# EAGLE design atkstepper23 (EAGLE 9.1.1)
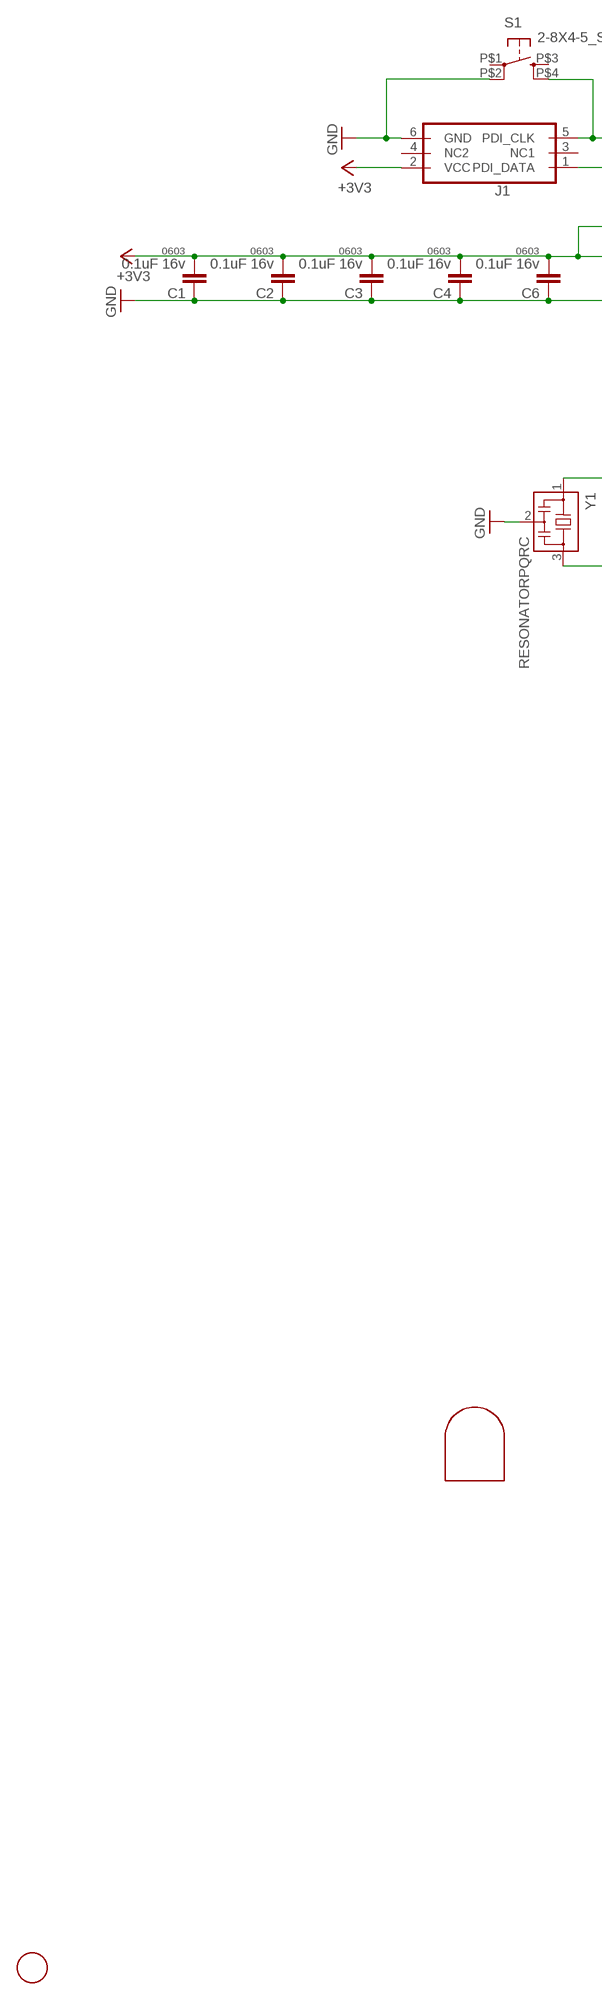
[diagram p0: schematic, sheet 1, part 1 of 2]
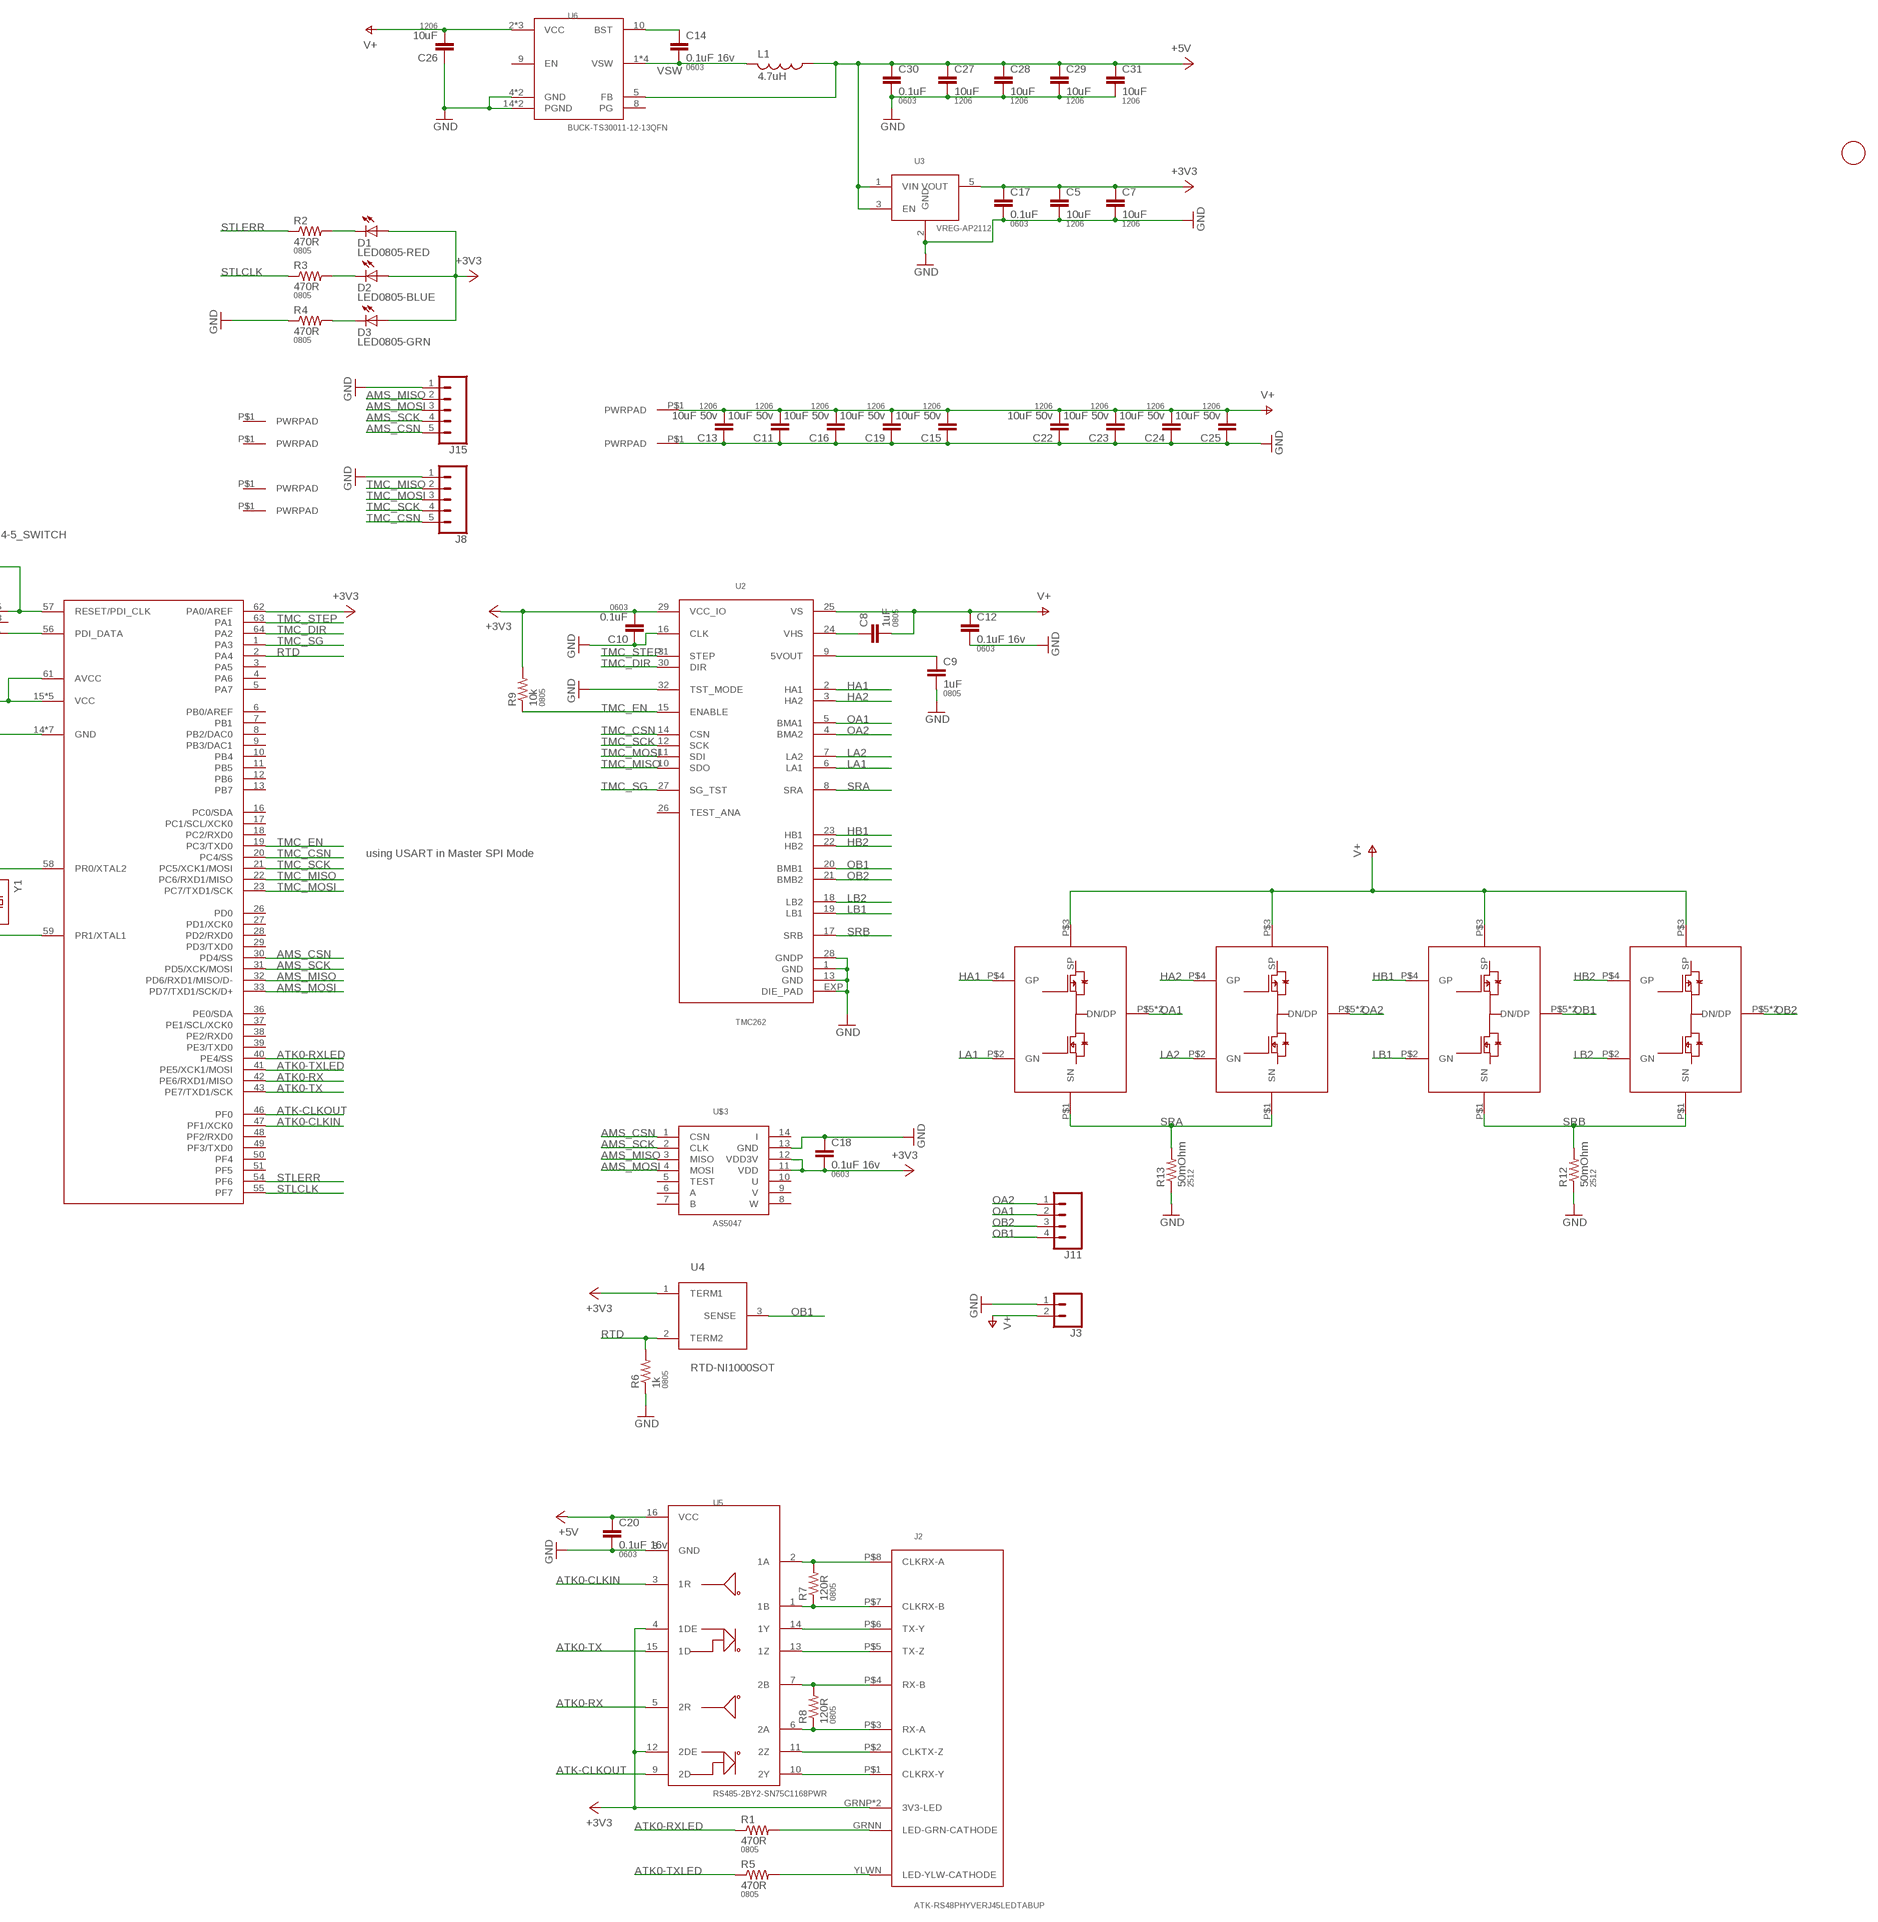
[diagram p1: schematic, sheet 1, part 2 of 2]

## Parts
C1  0.1uF 16v  CAP0603-CAP  [0603-CAP]
C2  0.1uF 16v  CAP0603-CAP  [0603-CAP]
C3  0.1uF 16v  CAP0603-CAP  [0603-CAP]
C4  0.1uF 16v  CAP0603-CAP  [0603-CAP]
C5  10uF  CAP1206  [1206]
C6  0.1uF 16v  CAP0603-CAP  [0603-CAP]
C7  10uF  CAP1206  [1206]
C8  1uF  CAP0805  [0805]
C9  1uF  CAP0805  [0805]
C10  0.1uF  CAP0603-CAP  [0603-CAP]
C11  10uF 50v  CAP1206  [1206]
C12  0.1uF 16v  CAP0603-CAP  [0603-CAP]
C13  10uF 50v  CAP1206  [1206]
C14  0.1uF 16v  CAP0603-CAP  [0603-CAP]
C15  10uF 50v  CAP1206  [1206]
C16  10uF 50v  CAP1206  [1206]
C17  0.1uF  CAP0603-CAP  [0603-CAP]
C18  0.1uF 16v  CAP0603-CAP  [0603-CAP]
C19  10uF 50v  CAP1206  [1206]
C20  0.1uF 16v  CAP0603-CAP  [0603-CAP]
C22  10uF 50v  CAP1206  [1206]
C23  10uF 50v  CAP1206  [1206]
C24  10uF 50v  CAP1206  [1206]
C25  10uF 50v  CAP1206  [1206]
C26  10uF  CAP1206  [1206]
C27  10uF  CAP1206  [1206]
C28  10uF  CAP1206  [1206]
C29  10uF  CAP1206  [1206]
C30  0.1uF  CAP0603-CAP  [0603-CAP]
C31  10uF  CAP1206  [1206]
D1  LED0805-RED  LED0805  [LED0805]
D2  LED0805-BLUE  LED0805  [LED0805]
D3  LED0805-GRN  LED0805  [LED0805]
J1  PDITHRU  [PDI_2X3_THRU]
J2  ATK-RS48PHYVERJ45LEDTABUP  [RJ45-LED-RJHSE-5381-UPTAB]
J3  CONN_02PTH3  [1X02_LONGPADS]
J4  PWRPADM3-SKINNY  [PWRPAD_3-25MM-SKINNY]
J6  PWRPADM3-SKINNY  [PWRPAD_3-25MM-SKINNY]
J8  CONN_05NO_SILK  [1X05_NO_SILK]
J9  PWRPADM3-STANDOFF  [PWRPAD_M3_STANDOFF]
J10  PWRPADM3-STANDOFF  [PWRPAD_M3_STANDOFF]
J11  CONN_04LONGPADS  [1X04_LONGPADS]
J12  PWRPADM3-SKINNY  [PWRPAD_3-25MM-SKINNY]
J13  PWRPADM3-SKINNY  [PWRPAD_3-25MM-SKINNY]
J15  CONN_05NO_SILK  [1X05_NO_SILK]
L1  4.7uH  INDUCTOR  [NRS5020T4R7MMGJ]
MP1  JRTOMBSTONE  [JRTOMBSTONE]
Q1  PNPAIR-STL40C30H3LL-FDD8424HSTM  [POWERFLAT-5X6]
Q2  PNPAIR-STL40C30H3LL-FDD8424HSTM  [POWERFLAT-5X6]
Q3  PNPAIR-STL40C30H3LL-FDD8424HSTM  [POWERFLAT-5X6]
Q4  PNPAIR-STL40C30H3LL-FDD8424HSTM  [POWERFLAT-5X6]
R1  470R  RESISTOR0805-RES  [0805]
R2  470R  RESISTOR0805-RES  [0805]
R3  470R  RESISTOR0805-RES  [0805]
R4  470R  RESISTOR0805-RES  [0805]
R5  470R  RESISTOR0805-RES  [0805]
R6  1k  RESISTOR0805-RES  [0805]
R7  120R  RESISTOR0805-RES  [0805]
R8  120R  RESISTOR0805-RES  [0805]
R9  10k  RESISTOR0805-RES  [0805]
R12  50mOhm  RESISTOR2512  [R2512]
R13  50mOhm  RESISTOR2512  [R2512]
S1  2-8X4-5_SWITCH  [TACT-SWITCH-KMR6]
U1  ATXMEGA_A3UQFN  [QFN-64-9X9MM]
U2  TMC262  [QFN32]
U3  VREG-AP2112  [SOT23-5]
U4  RTD-NI1000SOT  [SOT23]
U5  RS485-2BY2-SN75C1168PWR  [TSSOP16]
U6  BUCK-TS30011-12-13QFN  [QFN16-3X3-TI-RTE]
U$1  FIDUCIAL  [FIDUCIAL_1MM]
U$2  FIDUCIAL  [FIDUCIAL_1MM]
U$3  AS5047  [TSSOP14]
Y1  RESONATORPQRC  [RES_PRQC]

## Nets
+3V3: C1.2 C2.2 C3.2 C4.2 C5.1 C6.2 C7.1 C10.2 C17.1 C18.2 D1.1(A) D2.1(A) D3.1(A) J1.2(VCC) J2.GRNP(3V3-LED) J2.YLWP(3V3-LED) R9.2 U1.15(VCC) U1.25(VCC) U1.35(VCC) U1.45(VCC) U1.53(VCC) U1.61(AVCC) U1.62(PA0/AREF) U2.29(VCC_IO) U3.5(VOUT) U4.1(TERM1) U5.4(1DE) U5.12(2DE) U$3.11(VDD) U$3.12(VDD3V)
+5V: C20.1 C27.1 C28.1 C29.1 C30.1 C31.1 L1.1 U3.1(VIN) U3.3(EN) U5.16(VCC) U6.5(FB)
AMS_CSN: J15.5 U1.30(PD4/SS) U$3.1(CSN)
AMS_MISO: J15.2 U1.32(PD6/RXD1/MISO/D-) U$3.3(MISO)
AMS_MOSI: J15.3 U1.33(PD7/TXD1/SCK/D+) U$3.4(MOSI)
AMS_SCK: J15.4 U1.31(PD5/XCK/MOSI) U$3.2(CLK)
ATK0-CLKIN: U1.47(PF1/XCK0) U5.3(1R)
ATK0-RX: U1.42(PE6/RXD1/MISO) U5.5(2R)
ATK0-RXLED: R1.1 U1.40(PE4/SS)
ATK0-TX: U1.43(PE7/TXD1/SCK) U5.15(1D)
ATK0-TXLED: R5.1 U1.41(PE5/XCK1/MOSI)
ATK-CLKOUT: U1.46(PF0) U5.9(2D)
GND: C1.1 C2.1 C3.1 C4.1 C5.2 C6.1 C7.2 C9.2 C10.1 C11.1 C12.2 C13.1 C15.1 C16.1 C17.2 C18.1 C19.1 C20.2 C22.1 C23.1 C24.1 C25.1 C26.1 C27.2 C28.2 C29.2 C30.2 C31.2 J1.6(GND) J3.1 J8.1 J10.P$1(PWRPAD) J15.1 R4.1 R6.1 R12.1 R13.1 S1.P$2(P1) U1.14(GND) U1.24(GND) U1.34(GND) U1.44(GND) U1.52(GND) U1.60(GND) U1.P$1(GND) U2.1(GND) U2.13(GND) U2.16(CLK) U2.28(GNDP) U2.32(TST_MODE) U2.EXP(DIE_PAD) U3.2(GND) U5.8(GND) U6.4(GND) U6.14(PGND) U6.15(PGND) U6.TH(GND) U$3.13(GND) Y1.2
HA1: Q1.P$4(GP) U2.2(HA1)
HA2: Q2.P$4(GP) U2.3(HA2)
HB1: Q3.P$4(GP) U2.23(HB1)
HB2: Q4.P$4(GP) U2.22(HB2)
LA1: Q1.P$2(GN) U2.6(LA1)
LA2: Q2.P$2(GN) U2.7(LA2)
LB1: Q3.P$2(GN) U2.19(LB1)
LB2: Q4.P$2(GN) U2.18(LB2)
N$1: D3.2(C) R4.2
N$2: C8.1 U2.24(VHS)
N$3: J2.P$8(CLKRX-A) R7.2 U5.2(1A)
N$4: J1.5(PDI_CLK) S1.P$4(S1) U1.57(RESET/PDI_CLK)
N$5: D2.2(C) R3.2
N$6: D1.2(C) R2.2
N$7: U1.58(PR0/XTAL2) Y1.1
N$8: U1.59(PR1/XTAL1) Y1.3
N$10: J1.1(PDI_DATA) U1.56(PDI_DATA)
N$11: J2.P$7(CLKRX-B) R7.1 U5.1(1B)
N$12: J2.P$6(TX-Y) U5.14(1Y)
N$13: J2.P$5(TX-Z) U5.13(1Z)
N$14: J2.P$4(RX-B) R8.2 U5.7(2B)
N$15: J2.P$3(RX-A) R8.1 U5.6(2A)
N$16: J2.P$2(CLKTX-Z) U5.11(2Z)
N$17: J2.P$1(CLKRX-Y) U5.10(2Y)
N$18: C9.1 U2.9(5VOUT)
N$19: J2.GRNN(LED-GRN-CATHODE) R1.2
N$20: J2.YLWN(LED-YLW-CATHODE) R5.2
N$23: C14.1 U6.10(BST)
OA1: J11.2 Q1.P$5(DN/DP) Q1.P$8(DN/DP) U2.5(BMA1)
OA2: J11.1 Q2.P$5(DN/DP) Q2.P$8(DN/DP) U2.4(BMA2)
OB1: J11.4 Q3.P$5(DN/DP) Q3.P$8(DN/DP) U2.20(BMB1) U4.3(SENSE)
OB2: J11.3 Q4.P$5(DN/DP) Q4.P$8(DN/DP) U2.21(BMB2)
RTD: R6.2 U1.2(PA4) U4.2(TERM2)
SRA: Q1.P$1(SN) Q2.P$1(SN) R13.2 U2.8(SRA)
SRB: Q3.P$1(SN) Q4.P$1(SN) R12.2 U2.17(SRB)
STLCLK: R3.1 U1.55(PF7)
STLERR: R2.1 U1.54(PF6)
TMC_CSN: J8.5 U1.20(PC4/SS) U2.14(CSN)
TMC_DIR: U1.64(PA2) U2.30(DIR)
TMC_EN: R9.1 U1.19(PC3/TXD0) U2.15(ENABLE)
TMC_MISO: J8.2 U1.22(PC6/RXD1/MISO) U2.10(SDO)
TMC_MOSI: J8.3 U1.23(PC7/TXD1/SCK) U2.11(SDI)
TMC_SCK: J8.4 U1.21(PC5/XCK1/MOSI) U2.12(SCK)
TMC_SG: U1.1(PA3) U2.27(SG_TST)
TMC_STEP: U1.63(PA1) U2.31(STEP)
V+: C8.2 C11.2 C12.1 C13.2 C15.2 C16.2 C19.2 C22.2 C23.2 C24.2 C25.2 C26.2 J3.2 J9.P$1(PWRPAD) Q1.P$3(SP) Q2.P$3(SP) Q3.P$3(SP) Q4.P$3(SP) U2.25(VS) U6.2(VCC) U6.3(VCC) U6.11(VCC)
VSW: C14.2 L1.2 U6.1(VSW) U6.12(VSW) U6.13(VSW) U6.16(VSW)
Unconnected: J1.3(NC1) J1.4(NC2) J4.P$1(PWRPAD) J6.P$1(PWRPAD) J12.P$1(PWRPAD) J13.P$1(PWRPAD) S1.P$1(P) S1.P$3(S) U1.3(PA5) U1.4(PA6) U1.5(PA7) U1.6(PB0/AREF) U1.7(PB1) U1.8(PB2/DAC0) U1.9(PB3/DAC1) U1.10(PB4) U1.11(PB5) U1.12(PB6) U1.13(PB7) U1.16(PC0/SDA) U1.17(PC1/SCL/XCK0) U1.18(PC2/RXD0) U1.26(PD0) U1.27(PD1/XCK0) U1.28(PD2/RXD0) U1.29(PD3/TXD0) U1.36(PE0/SDA) U1.37(PE1/SCL/XCK0) U1.38(PE2/RXD0) U1.39(PE3/TXD0) U1.48(PF2/RXD0) U1.49(PF3/TXD0) U1.50(PF4) U1.51(PF5) U2.26(TEST_ANA) U6.8(PG) U6.9(EN) U$3.5(TEST) U$3.6(A) U$3.7(B) U$3.8(W) U$3.9(V) U$3.10(U) U$3.14(I)

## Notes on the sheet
- using USART in Master SPI Mode

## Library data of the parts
C1-C4 C6 C10 C12 C14 C17 C18 C20 C30 = borkedlabs-passives:CAP: Capacitor; PACKAGE: 0603
C5 C7 C11 C13 C15 C16 C19 C22-C29 C31 = borkedlabs-passives:CAP: Capacitor; PACKAGE: 1206
C8 C9 = borkedlabs-passives:CAP: Capacitor; PACKAGE: 0805
D1-D3 = lights:LED: LED
J1 = microcontrollers:PDI: Multi connection point. Often used as Generic Header-pin footprint for 0.1 inch spaced/style header connections You can populate with any combo of single row headers, but if you'd like an exact match, check these: Header - 2x3 (Male, 0.1") (PRT-12807) Header - 2x3 (Female, 0.1") (PRT-13010) 2x3 Pin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
J2 = connector:ATK-RS48PHYVE
J3 = SparkFun-Connectors:CONN_02: Multi connection point. Often used as Generic Header-pin footprint for 0.1 inch spaced/style header connections
J4 J6 J9 J10 J12 J13 = power:PWRPAD
J8 J15 = SparkFun-Connectors:CONN_05: Multi connection point. Often used as Generic Header-pin footprint for 0.1 inch spaced/style header connections On any of the 0.1 inch spaced packages, you can populate with these: Break Away Headers - Straight (PRT-00116) Break Away Male Headers - Right Angle (PRT-00553) Female Headers (PRT-00115)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
J11 = SparkFun-Connectors:CONN_04: Multi connection point. Often used as Generic Header-pin footprint for 0.1 inch spaced/style header connections On any of the 0.1 inch spaced packages, you can populate with these: Break Away Headers - Straight (PRT-00116) Break Away Male Headers - Right Angle (PRT-00553) Female Headers (PRT-00115)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; PROD_ID: CONN-09696
L1 = power:INDUCTOR
MP1 = connector:JRTOMBSTONE
Q1-Q4 = power:PNPAIR-STL40C30H3LL-FDD8424H
R1-R9 = borkedlabs-passives:RESISTOR: Resistor; PACKAGE: 0805
R12 R13 = borkedlabs-passives:RESISTOR: Resistor; PACKAGE: 2512
S1 = fab:2-8X4-5_SWITCH
U1 = microcontrollers:ATXMEGA_A3U
U2 = power:TMC262
U3 = power:VREG-AP2112
U4 = sensor:RTD-NI1000SOT
U5 = comm:RS485-2BY2-SN75C1168PWR
U6 = power:BUCK-TS30011-12-13
U$1 U$2 = connector:FIDUCIAL: For use by pick and place machines to calibrate the vision/machine, 1mm
U$3 = sensor:AS5047
Y1 = passives:RESONATOR

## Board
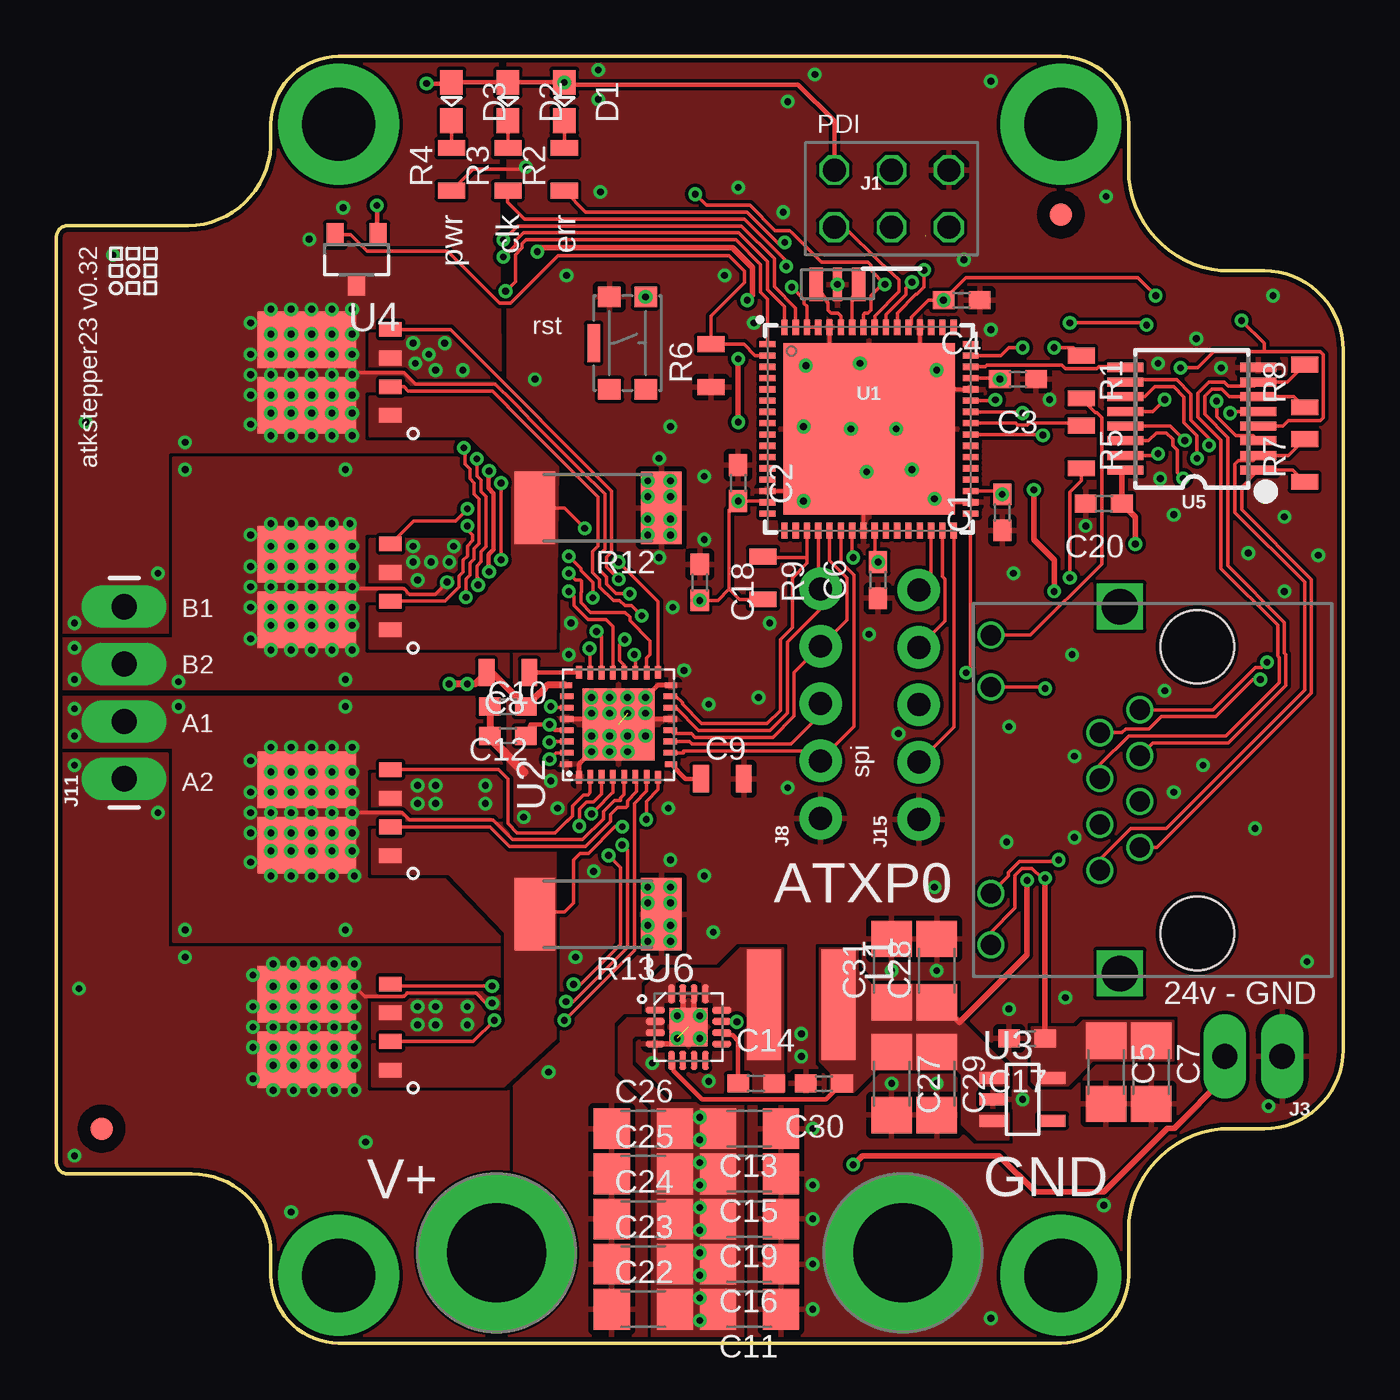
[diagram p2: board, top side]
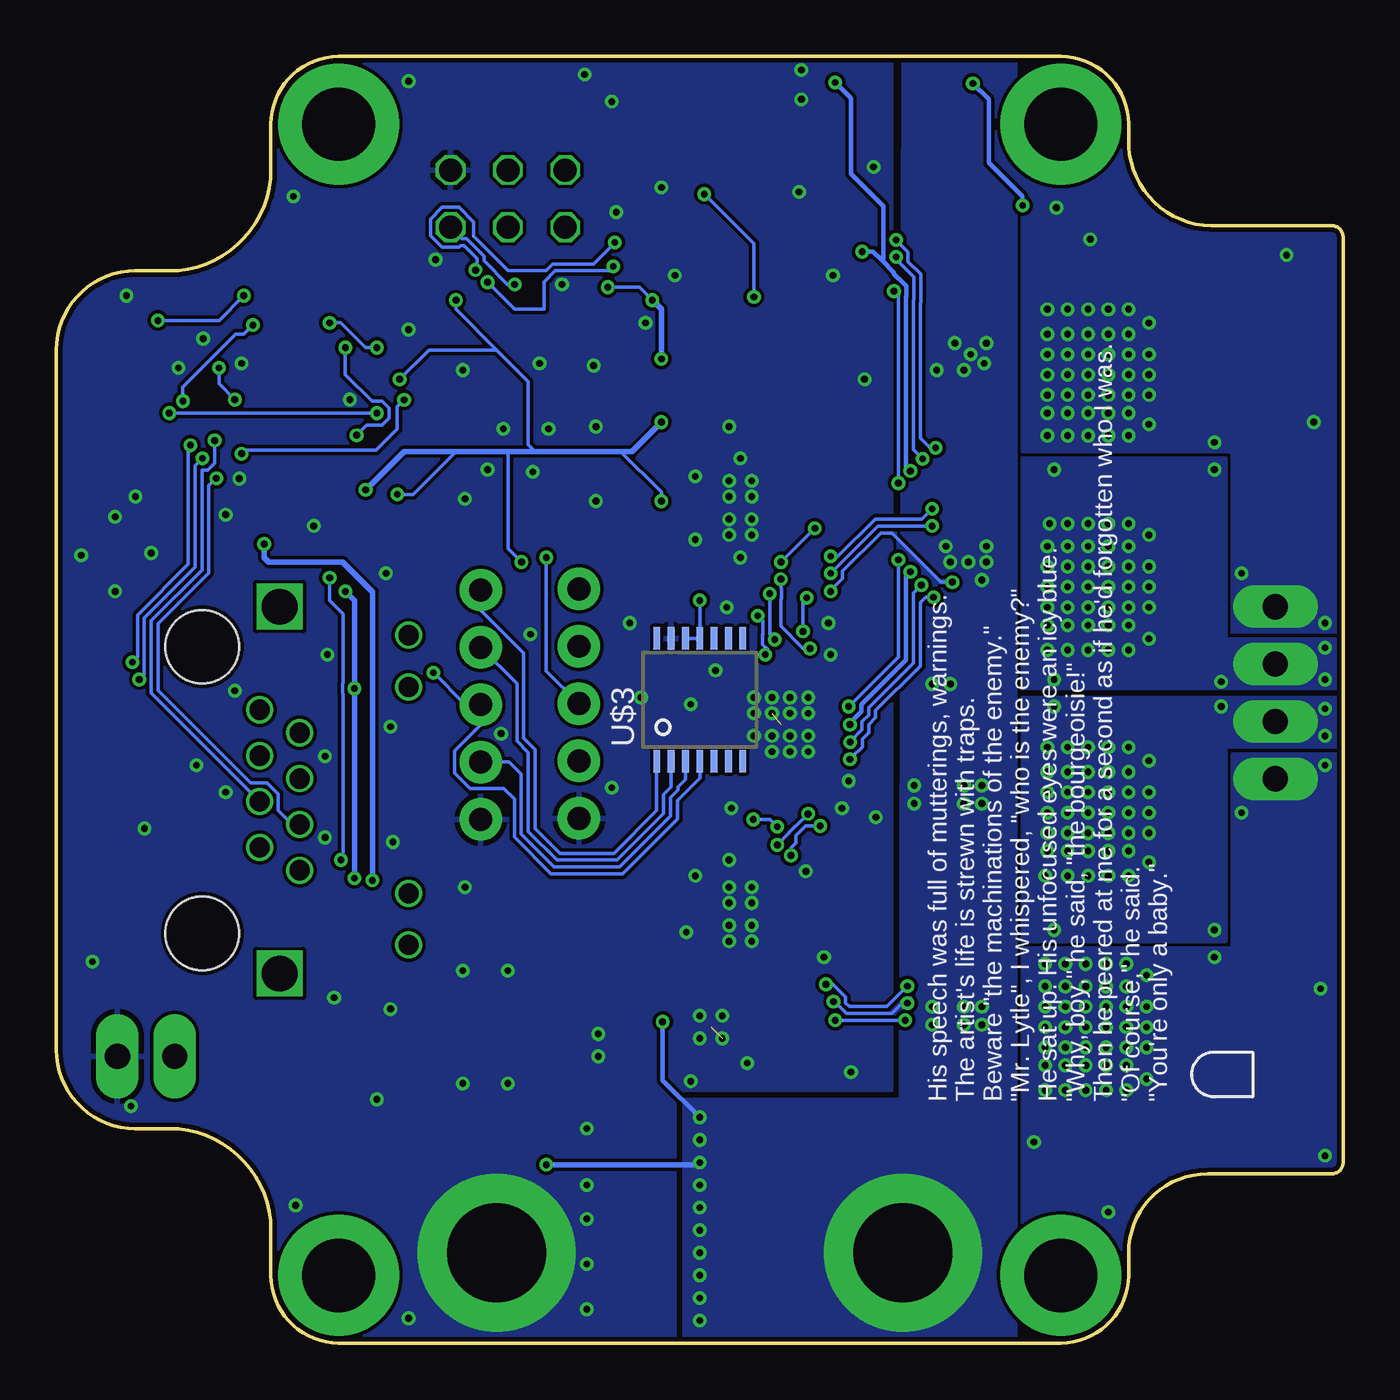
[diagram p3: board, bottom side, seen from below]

Size 57 x 57 mm. Coordinates in mm from the lower left corner, seen from the top.
Outline: 44.5,0 12.5,0 arc-90 9.5,3 9.5,4 arc90 6,7.5 0.5,7.5 arc-90 0,8 0,49 arc-90 0.5,49.5 5.5,49.5 arc90 9.5,53 9.5,54 arc-90 12.5,57 44.5,57 arc-90 47.5,54 47.5,52 arc90 52,47.5 53.5,47.5 arc-90 57,44 57,13 arc-90 53.5,9.5 52,9.5 arc90 47.5,5 47.5,3 arc-90 44.5,0
Copper layers (1*16): Top 0.035mm / dielectric 1.5mm / Bottom 0.035mm
Design rules "default *": minimum track width 6mil, minimum drill 0.3mm, track to track 6mil, track to pad 6mil, pad to pad 6mil, via to via 6mil, smd to smd 6mil, copper to edge 8mil, drill to drill 8mil, minimum pad ring 6mil, minimum via ring 6mil, stop-mask expansion 4mil, vias tented up to drill 27mil, thermal gap 9mil

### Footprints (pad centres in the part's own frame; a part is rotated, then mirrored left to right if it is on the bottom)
0603-CAP = smd 0.96 x 0.8: 1 -0.8,0; 2 0.8,0
1206 = smd 1.6 x 1.8: 1 -1.4,0; 2 1.4,0
0805 = smd 0.7 x 1.2: 1 -0.95,0; 2 0.95,0
LED0805 = smd 1.1 x 1: 1 -0.85,0; 2 0.85,0
PDI_2X3_THRU = drill 1.016 octagon: 1 -2.54,-1.27; 2 -2.54,1.27; 3 0,-1.27; 4 0,1.27; 5 2.54,-1.27; 6 2.54,1.27
RJ45-LED-RJHSE-5381-UPTAB = drill 0.889: GRNN 6.858,6.604; GRNP 4.572,6.604; YLWN -4.572,6.604; YLWP -6.858,6.604 | drill 0.9: P$1 3.556,0; P$2 2.54,1.778; P$3 1.524,0; P$4 0.508,1.778; P$5 -0.508,0; P$6 -1.524,1.778; P$7 -2.54,0; P$8 -3.556,1.778 | drill 1.575 square: SHDL1 -8.128,0.889; SHDL2 8.128,0.889 | hole 3.251: -6.35,-2.54; 6.35,-2.54
1X02_LONGPADS = drill 1.118 pad 1.88 long: 1 0,0; 2 2.54,0
PWRPAD_3-25MM-SKINNY = drill 3.25 pad 5.35: P$1 0,0
1X05_NO_SILK = drill 1.016 pad 1.88: 1 0,0; 2 2.54,0; 3 5.08,0; 4 7.62,0; 5 10.16,0
PWRPAD_M3_STANDOFF = drill 4.4 pad 7: P$1 0,0
1X04_LONGPADS = drill 1.118 pad 1.88 long: 1 0,0; 2 2.54,0; 3 5.08,0; 4 7.62,0
NRS5020T4R7MMGJ = smd 4.9 x 1.5: 1 0,1.65; 2 0,-1.65
POWERFLAT-5X6 = smd 0.65 x 1: P$1 -1.905,-2.8; P$2 -0.635,-2.8; P$3 0.635,-2.8; P$4 1.905,-2.8 | smd 2.5 x 4.35: P$5 1.45,0.9; P$8 -1.45,0.9
R2512 = smd 1.8 x 3.2: 1 -2.8,0; 2 2.8,0
TACT-SWITCH-KMR6 = smd 0.9 x 1: P$1 -2.05,0.8; P$2 2.05,0.8; P$3 -2.05,-0.8; P$4 2.05,-0.8 | smd 1.7 x 0.55: P$5 0,1.5
QFN-64-9X9MM = smd 0.7 x 0.275: 1 -4.5,3.75; 2 -4.5,3.25; 3 -4.5,2.75; 4 -4.5,2.25; 5 -4.5,1.75; 6 -4.5,1.25; 7 -4.5,0.75; 8 -4.5,0.25; 9 -4.5,-0.25; 10 -4.5,-0.75; 11 -4.5,-1.25; 12 -4.5,-1.75; 13 -4.5,-2.25; 14 -4.5,-2.75; 15 -4.5,-3.25; 16 -4.5,-3.75; 33 4.5,-3.75; 34 4.5,-3.25; 35 4.5,-2.75; 36 4.5,-2.25; 37 4.5,-1.75; 38 4.5,-1.25; 39 4.5,-0.75; 40 4.5,-0.25; 41 4.5,0.25; 42 4.5,0.75; 43 4.5,1.25; 44 4.5,1.75; 45 4.5,2.25; 46 4.5,2.75; 47 4.5,3.25; 48 4.5,3.75 | smd 0.275 x 0.7: 17 -3.75,-4.5; 18 -3.25,-4.5; 19 -2.75,-4.5; 20 -2.25,-4.5; 21 -1.75,-4.5; 22 -1.25,-4.5; 23 -0.75,-4.5; 24 -0.25,-4.5; 25 0.25,-4.5; 26 0.75,-4.5; 27 1.25,-4.5; 28 1.75,-4.5; 29 2.25,-4.5; 30 2.75,-4.5; 31 3.25,-4.5; 32 3.75,-4.5; 49 3.75,4.5; 50 3.25,4.5; 51 2.75,4.5; 52 2.25,4.5; 53 1.75,4.5; 54 1.25,4.5; 55 0.75,4.5; 56 0.25,4.5; 57 -0.25,4.5; 58 -0.75,4.5; 59 -1.25,4.5; 60 -1.75,4.5; 61 -2.25,4.5; 62 -2.75,4.5; 63 -3.25,4.5; 64 -3.75,4.5 | smd 7.6 x 7.6: P$1 0,0
QFN32 = smd 0.55 x 0.25: 1 -2.325,1.75; 8 -2.325,-1.75; 17 2.325,-1.75; 24 2.325,1.75 | smd 0.6 x 0.25: 2 -2.3,1.25; 3 -2.3,0.75; 4 -2.3,0.25; 5 -2.3,-0.25; 6 -2.3,-0.75; 7 -2.3,-1.25; 18 2.3,-1.25; 19 2.3,-0.75; 20 2.3,-0.25; 21 2.3,0.25; 22 2.3,0.75; 23 2.3,1.25 | smd 0.25 x 0.55: 9 -1.75,-2.325; 16 1.75,-2.325; 25 1.75,2.325; 32 -1.75,2.325 | smd 0.25 x 0.6: 10 -1.25,-2.3; 11 -0.75,-2.3; 12 -0.25,-2.3; 13 0.25,-2.3; 14 0.75,-2.3; 15 1.25,-2.3; 26 1.25,2.3; 27 0.75,2.3; 28 0.25,2.3; 29 -0.25,2.3; 30 -0.75,2.3; 31 -1.25,2.3 | smd 3.2 x 3.2: EXP 0,0
SOT23-5 = smd 0.533 x 1.194: 1 -0.95,-1.306; 2 0,-1.306; 3 0.95,-1.306; 4 0.95,1.306; 5 -0.95,1.306
SOT23 = smd 0.762 x 1.016: 1 -0.95,-1.1; 2 0.95,-1.1; 3 0,1.1
TSSOP16 = smd 0.4 x 1.6: 1 -2.225,-2.85; 2 -1.575,-2.85; 3 -0.925,-2.85; 4 -0.275,-2.85; 5 0.375,-2.85; 6 1.025,-2.85; 7 1.675,-2.85; 8 2.325,-2.85; 9 2.325,3.05; 10 1.675,3.05; 11 1.025,3.05; 12 0.375,3.05; 13 -0.275,3.05; 14 -0.925,3.05; 15 -1.575,3.05; 16 -2.225,3.05
QFN16-3X3-TI-RTE = smd 0.85 x 0.3: 1 -1.475,0.75; 2 -1.475,0.25; 3 -1.475,-0.25; 4 -1.475,-0.75; 9 1.475,-0.75; 10 1.475,-0.25; 11 1.475,0.25; 12 1.475,0.75 | smd 0.3 x 0.85: 5 -0.75,-1.475; 6 -0.25,-1.475; 7 0.25,-1.475; 8 0.75,-1.475; 13 0.75,1.475; 14 0.25,1.475; 15 -0.25,1.475; 16 -0.75,1.475 | smd 1.7 x 1.7: TH 0,0
FIDUCIAL_1MM = smd 1 x 1: 1 0,0
TSSOP14 = smd 0.305 x 0.991: 1 -1.905,-2.718; 2 -1.27,-2.718; 3 -0.635,-2.718; 4 0,-2.718; 5 0.635,-2.718; 6 1.27,-2.718; 7 1.905,-2.718; 8 1.905,2.718; 9 1.27,2.718; 10 0.635,2.718; 11 0,2.718; 12 -0.635,2.718; 13 -1.27,2.718; 14 -1.905,2.718
RES_PRQC = smd 0.6 x 1.5: 1 -0.95,0; 3 0.95,0 | smd 0.4 x 1.5: 2 0,0

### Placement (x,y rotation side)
C1  41.9,36.8 90 top
C2  30.2,38.1 270 top
C3  42.6,42.7 180 top
C4  40.1,46.2 180 top
C5  46.5,12 270 top
C6  36.4,33.8 90 top
C7  48.5,12 270 top
C8  20,29.7 180 top
C9  29.5,25 0 top
C10  20,26.9 0 top
C11  30.7,1.5 180 top
C12  20,28.2 180 top
C13  30.7,9.5 180 top
C14  31,11.5 0 top
C15  30.7,7.5 180 top
C16  30.7,3.5 180 top
C17  43,13.5 180 top
C18  28.5,33.7 270 top
C19  30.7,5.5 180 top
C20  46.4,37.2 180 top
C22  26,1.5 0 top
C23  26,3.5 0 top
C24  26,5.5 0 top
C25  26,7.5 0 top
C26  26,9.5 0 top
C27  37,11.5 270 top
C28  39,16.5 90 top
C29  39,11.5 270 top
C30  34,11.5 180 top
C31  37,16.5 90 top
D1  22.5,55 270 top
D2  20,55 270 top
D3  17.5,55 270 top
J1  37,50.7 0 top
J2  48,24.5 90 top
J3  54.3,12.7 180 top
J4  12.5,3 180 top
J6  44.5,3 180 top
J8  33.85,23.25 90 top
J9  19.5,4 180 top
J10  37.5,4 180 top
J11  3,25 90 top
J12  12.5,54 180 top
J13  44.5,54 180 top
J15  38.2,23.2 90 top
L1  33,15 270 top
MP1  5,11.9 90 bottom
Q1  12,23.5 90 top
Q2  12,14 90 top
Q3  12,43 90 top
Q4  12,33.5 90 top
R1  45.4,42.8 270 top
R2  22.5,52 90 top
R3  20,52 90 top
R4  17.5,52 90 top
R5  45.4,39.7 270 top
R6  29,43.3 90 top
R7  55.3,39.1 90 top
R8  55.3,42.4 90 top
R9  31.3,33.9 270 top
R12  24,37 180 top
R13  24,19 180 top
S1  25.3,44.3 90 top
U1  36,40.5 0 top
U2  24.9,27.4 90 top
U3  42.8,10.8 270 top
U4  13.3,48 180 top
U5  50.4,40.9 90 top
U6  28,14 0 top
U$1  2,9.5 0 top
U$2  44.5,50 0 top
U$3  28.5,28.5 0 bottom
U$5  [CBA-SILK-LOGO]  3.4,47.5 90 top
Y1  34.6,46.9 180 top

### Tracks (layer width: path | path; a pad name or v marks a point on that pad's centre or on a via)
+3V3  (via drill 0.3)
  Top 0.152: v32.58,46.77 33.12,46.23 33.12,46.05 33.25,45.93 U1.62 U1.61 | U1.53 37.88,45.13 37.88,45.45 38.64,46.2 C4.2 40.3,47.2 47.9,47.2 v48.7,46.4 | C3.2 41.75,42.75 U1.45 | U1.35 41.75,37.75 C1.2 | C6.2 36.25,34.75 U1.25 | U1.15 31.45,37.3 C2.2 29.8,36.9 29.8,33.4 | 29.8,33.4 29.3,32.9 C18.2 | 29.8,33.4 30.25,32.95 R9.2 | U5.12 48.58,41.27 v49.1,41.8 | v49.8,43.21 50.55,43.21 51.28,43.93 53.5,43.93 | 53.5,43.93 55.99,43.93 56.13,43.8 56.13,41.01 55.99,40.87 54.57,40.87 54.33,40.62 U5.4 | v52.5,45.3 53.5,44.3 53.5,43.93 | J2.YLWP 41.4,18.2 42.47,19.27 42.47,20.72 42.78,21.03 43.22,21.03 43.65,20.6 v43.8,20.6 | J2.GRNP 43.73,29.07 v43.8,29
  Top 0.203: U2.29 22.09,27.15 v21.84,27.4 21,27.4 C10.2 | v19.16,34.16 19.16,34.45 19.14,34.47 19.14,34.93 19.37,35.16 19.37,37.64 19.14,37.87 19.14,38.33 19.16,38.35 v19.16,38.63 | v16.4,55.8 17.45,55.8 D3.1 D2.1 D1.1 22.6,55.75 32.86,55.75 34.46,54.15 J1.2 | v14.2,50.4 14.2,49.15 U4.1
  Top 0.254: v30.2,40.8 v30.2,43.6 | v30.6,46.2 30.84,46.44 30.84,47.64 29.95,48.52 21.48,48.52 v21.3,48.35 | C17.1 v43.8,20.6 | v44.2,33.3 44.2,34.7 43.3,35.6 v43.3,37.8
  Bottom 0.152: v32.58,46.77 31.18,46.77 v30.6,46.2 | 35.8,39.5 36.1,39.8 36.1,42.6 37.5,44 | 37.5,44 39.3,45.8 C4.2 | 37.5,44 40.5,44 C3.2 | 39.3,39.5 41.2,37.6 C1.2 | 37,39.5 37,35.2 C6.2 | 32,39.5 30.2,37.7 C2.2 | C18.2 U$3.11 U$3.12 | v49.1,41.8 49.8,42.5 v49.8,43.21 | v48.7,46.4 49.8,45.3 v52.5,45.3
  Bottom 0.203: v21.84,27.4 21.84,27.47 21.34,27.97 21.34,28.29 19.37,30.26 19.37,33.96 v19.16,34.16 | v19.16,38.63 19.37,38.84 19.37,46.34 19.34,46.37 19.34,46.83 19.67,47.16 19.7,47.16 19.9,47.36 19.9,47.43 20.44,47.96 | D1.1 21.8,55.15 21.8,51.8 20.36,50.36 20.36,48.04 20.44,47.96 | v16.4,55.8 15.7,55.1 15.7,52.3 14.2,50.8 v14.2,50.4 | v21.3,48.35 20.82,48.35 20.44,47.96
  Bottom 0.254: v43.3,37.8 41.6,39.5 39.3,39.5 37,39.5 35.8,39.5 32,39.5 31.5,39.5 v30.2,40.8 | v30.2,43.6 30.2,45.8 v30.6,46.2 | v43.8,20.6 v43.8,29 43.8,32.9 v44.2,33.3
  other vias: 22.5,55.85 39.3,46.2 41.8,42.7 41.9,37.6 36.4,34.6 30.2,37.3 28.5,32.9
  pour Top (no thermals): 43.2,14 43.2,11.6 43.4,11.4 44.8,11.4 45.9,12.5 49.5,12.5 49.5,14.3 45.5,14.3 45.2,14
+5V  (via drill 0.3)
  Top 0.203: U6.5 27.35,12.43 27.35,12.06 28.61,10.8 34.1,10.8 C30.1
  Top 0.254: v47.8,35.4 47.8,36.6 C20.1 47.2,38.52 U5.16 | v43,20.5 43,17.2 40,14.2 39.1,15.1 C28.1
  Bottom 0.254: v47.8,35.4 47.8,34.8 47.6,34.6 44.32,34.6 43,33.28 v43,20.5
  pour Top (no thermals): 33.8,17.5 33.8,12.5 34.3,12 34.3,11.1 35.3,11.1 36.3,12.1 36.4,12.1 39.9,12.1 40.1,11.9 40.1,9.7 40.8,9 42.2,9 42.2,10.2 40.8,10.2 40.8,11.4 42.2,11.4 42.2,11.9 42.2,12.2 39.9,14.5 39.9,15.9 36.1,15.9 35.5,16.5 35.5,16.6 35.5,17.5
AMS_CSN
  Top 0.152: U1.30 38.75,33.91 J15.5
  Bottom 0.152: U$3.1 30.41,23.59 32.3,21.7 34.7,21.7 35.8,22.8 35.8,26.3 36.3,26.8 36.3,30.57 38.2,32.47 J15.5
AMS_MISO
  Top 0.152: U1.32 39.75,27.29 J15.2
  Bottom 0.152: J15.2 36.94,25.74 36.41,25.21 36.41,22.55 34.95,21.09 32.05,21.09 29.8,23.34 29.8,24.17 29.46,24.5 29.46,24.64 29.14,24.96 U$3.3
AMS_MOSI  (via drill 0.3)
  Top 0.152: U1.33 40.5,29.9 v40.3,29.7
  Bottom 0.152: J15.3 | U$3.4 28.5,25.04 29.49,24.05 29.49,23.22 31.92,20.79 35.08,20.79 36.71,22.42 36.71,24.1 37.19,24.57 38.68,24.57 39.37,25.26 39.37,26.22 38.21,27.38 J15.3 | v40.3,29.7 38.89,28.29 J15.3
AMS_SCK
  Top 0.152: U1.31 39.25,33.96 39.37,33.84 39.37,31.99 J15.4
  Bottom 0.152: U$3.2 29.77,24.63 30.1,24.3 30.1,23.47 32.17,21.39 34.83,21.39 36.1,22.67 36.1,26.17 36.6,26.67 36.6,29.22 J15.4
ATK0-CLKIN  (via drill 0.3)
  Top 0.152: U5.3 53.03,40.2 52.25,40.2 51.4,41.05 v51.4,41.73 | v42.8,44.1 42.2,44.1 41.85,43.75 U1.47 | v44.9,45.2 48.2,45.2 v48.3,45.1
  Bottom 0.152: v42.8,44.1 43.3,44.1 44.4,45.2 v44.9,45.2 | v51.4,41.73 51.4,42.36 49.06,44.7 48.7,44.7 v48.3,45.1
ATK0-RX  (via drill 0.3)
  Top 0.152: U1.42 42.75,41.25 v42.8,41.2 | v52,41.2 52.08,41.27 U5.5
  Bottom 0.152: v42.8,41.2 v52,41.2
ATK0-RXLED  (via drill 0.3)
  Top 0.152: U1.40 43.67,40.25 v43.7,40.22 | v44.2,44.1 45.05,44.1 R1.1
  Bottom 0.152: v43.7,40.22 43.25,40.67 42.58,40.67 42.27,40.98 42.27,41.42 42.58,41.73 43.02,41.73 44.2,42.91 v44.2,44.1
ATK0-TX  (via drill 0.3)
  Top 0.152: U1.43 41.57,41.75 v41.6,41.78 | v48.8,39.4 48.73,39.33 U5.15
  Bottom 0.152: v41.6,41.78 41.9,41.48 41.9,40.5 42.84,39.55 48.65,39.55 v48.8,39.4
ATK0-TXLED
  Top 0.152: R5.1 45.3,40.75 43.1,40.75 43.02,40.67 42.58,40.67 42.5,40.75 U1.41
ATK-CLKOUT
  Top 0.152: U5.9 47.33,43.25 46.17,43.25 46.09,43.17 44.7,43.17 44.55,43.33 41.23,43.33 41.15,43.25 U1.46
GND  (via drill 0.3)  (2 unrouted)
  Top 0.152: U1.60 34.25,42.25 35.9,40.6 35.75,40.45 35.75,40.4 33.1,37.75 U1.14 | U1.52 38.25,42.75 36.05,40.55 36.95,39.65 | 36.95,39.65 v35.9,38.6 35.75,38.75 U1.24 | U1.34 39.35,37.25 36.95,39.65 | U1.44 39.85,42.25 v39,43.1 | R4.1 18.45,52 20.5,52
  Top 0.203: U2.1 23.15,25.65 v23.7,26.2 | U2.13 26.35,27.65 v26.1,27.9 | U2.16 26.65,29.15 v26.1,28.6 | U2.28 23.45,27.65 v23.7,27.9
  Top 0.254: U6.15 27.75,14.75 v27.5,14.5 | U6.14 28.25,14.75 v28.5,14.5 | U6.4 27.25,13.25 v27.5,13.5
  Top 0.305: C12.2 C10.1
  Top 0.406: C10.1 19.2,26.8 20.7,25.3
  other vias: 24.5,26.2 25.3,26.2 26.1,26.9 23.7,26.9 24.5,26.9 25.3,26.9 24.5,27.9 25.3,27.9 23.7,28.6 24.5,28.6 25.3,28.6 27.2,17.8 27.2,18.5 27.2,19.5 27.2,20.2 27.2,21.4 27.2,35.8 27.2,36.5 27.2,37.5 27.2,38.2 28.7,38.4 28.7,35.6 27.8,29.8 28.9,28.3 21.2,42.7 29.6,47.3 22.6,47.3 27.1,23.7 41.4,1.1 20.7,23.3 21.9,24.9 22.2,23.7 27.3,32.6 27.2,40.6 34.6,46.9 33.2,43.3 38.9,37.4 33.1,37.3 31.6,31.9 26.2,18.5 26.2,19.5 28.7,20.7 26.2,17.8 26.2,20.2 26.2,35.8 26.2,36.5 26.2,37.5 26.2,38.2 26.7,39.2 26.7,34.8 22.8,31.9 22.7,30.5 23,17.1 23.8,20.9 50.5,44.5 48.8,43.4 51.6,43.2 30.9,45.2 44,41.8 33.1,40.6 37.2,40.5 35.6,43.4 37.9,38.7 35.2,40.5 33.5,9.5 33.5,7 33.5,5.5 33.5,3.5 33.5,1.5 46.4,6.1 53.7,10.5 55.4,16.9 42.4,34.1 45.6,36.2 48.9,38.3 53.5,37.5 53.9,46.4 41.4,44.9 40.2,48 46.5,50.8 41.4,55.9 24,56.4 24,55.1 20.8,52.1 24.1,51 28.5,13.5 28.9,11.6 26.4,12.4 33,12.7 33,13.7 37,11.5 39,11.5 37,16.5 39,16.5 42.8,10.8 42.1,22.2 45.1,22.4 45.1,26 42.2,27.3 45,30.5 52.8,35 54.4,33.3 50.8,25.6 49.5,24.4 49.1,28.9 49.5,36.7 54.4,36.6 55.9,34.9 53.1,22.8 44.7,15.3 42.2,14.8 38.9,20.2 29.1,18.2 21.8,12 30.2,51.2 32.2,50.1 32.4,55 33.6,56.2 32.4,24.6 31.1,28.6 37.3,27 36,31.4
  pour Bottom: 29.6,-0.5 29.6,11.2 20,11.2 20,59.5 59.5,59.5 59,-0.5
  pour Top (rank 6): 20,60.5 20,-2 61,-2 61,60.5
HA1
  Top 0.152: U2.2 23.65,24.39 23.54,24.28 23.36,24.28 22.86,23.79 22.86,23.36 22.64,23.13 22.64,23.14 22.1,22.61 20.4,22.61 20,23.01 20,25 19.59,25.41 Q1.P$4
HA2  (via drill 0.3)
  Top 0.152: v22.91,15.89 23.23,15.89 24.99,17.65 24.99,21.07 v24.46,21.6 | v23.17,22.91 23.17,23.66 23.48,23.98 23.8,23.98 24.15,24.32 U2.3 | v19.3,15.81 14.89,15.81 Q2.P$4
  Bottom 0.152: v19.3,15.81 20.2,14.91 21.87,14.91 22.04,15.08 22.04,15.35 22.59,15.89 v22.91,15.89 | v24.46,21.6 24.46,21.94 24.23,22.16 24.23,22.48 23.81,22.91 v23.17,22.91
HB1  (via drill 0.3)
  Top 0.152: v24.91,33.84 24.37,34.38 24.37,34.82 24.6,35.05 | 24.6,35.05 | 24.6,35.05 24.6,37.74 21.45,40.89 21.45,40.92 20.54,41.83 20.44,41.92 20.44,41.93 17.46,44.91 Q3.P$4 | U2.23 23.65,30.74 v23.62,30.77
  Bottom 0.152: v24.91,33.84 24.91,33.46 24.87,33.42 24.87,32.98 24.91,32.94 24.91,31.75 23.92,30.77 v23.62,30.77
HB2  (via drill 0.3)
  Top 0.152: v18.2,36.96 v18.2,36.95 17.67,36.42 15.82,36.42 Q4.P$4 | v22.7,34.86 v22.7,34.85 23.23,34.32 23.23,34.23 23.76,33.69 v23.76,33.02 | v23.93,31.53 24.15,31.31 U2.22
  Bottom 0.152: v18.2,36.96 18.66,36.51 20.73,36.51 22.42,34.82 22.66,34.82 v22.7,34.86 | v23.93,31.53 23.93,32.85 v23.76,33.02
LA1
  Top 0.152: U2.6 25.7,25.05 25.7,24.43 25.3,24.03 25.3,23.8 25.23,23.73 24.85,23.73 24.54,23.42 24.54,23.1 23.44,22 20.07,22 19.21,22.86 Q1.P$2
LA2  (via drill 0.3)
  Top 0.152: v22.5,14.3 25.6,17.4 25.6,23.9 26.15,24.45 U2.7 | Q2.P$2 18.46,13.37 v19.4,14.3
  Bottom 0.152: v19.4,14.3 v22.5,14.3
LB1  (via drill 0.3)
  Top 0.152: U2.19 25.65,30.45 v25.6,30.5 | v25.93,32.22 25.48,32.67 25.18,32.67 24.95,32.9 24.67,32.9 24.07,33.5 24.07,33.82 23.76,34.13 23.76,35.07 23.99,35.3 23.99,37.48 20.01,41.46 20.01,41.49 19.32,42.18 15.59,42.18 15.4,42.37 Q3.P$2
  Bottom 0.152: v25.6,30.5 25.5,30.6 25.5,30.74 25.71,30.95 25.71,31.39 25.7,31.4 25.7,31.99 v25.93,32.22
LB2  (via drill 0.3)
  Top 0.152: v18.2,36.2 18.2,36.03 18.43,35.8 18.43,35.55 18.2,35.32 18.2,34.87 18.02,34.69 18.02,34.16 17.84,33.97 17.84,33.49 17.21,32.87 Q4.P$2 | U2.18 26.15,30.35 26.3,30.5 26.3,31.1 25.4,32 25.4,32.16 25.2,32.36 23.67,32.36 23.23,32.8 23.23,33.24 23.26,33.27 23.26,33.76 23.23,33.8 23,33.8 v22.7,34.1
  Bottom 0.152: v18.2,36.2 20.6,36.2 v22.7,34.1
N$1
  Top 0.152: D3.2 R4.2
N$2
  Top 0.203: U2.24 23.12,29.7 C8.1
N$3
  Top 0.152: R7.2 54.58,39.33 U5.2 53.03,39.1 52.35,39.1 52.2,38.95 52.2,36.8 55.3,33.71 55.3,28.93 49.17,22.8 47.6,22.8 46.22,21.42 J2.P$8
N$4  (via drill 0.3)
  Top 0.152: U1.57 35.75,45.57 35.8,45.62 35.95,45.62 36.08,45.76 36.08,46.4 36.58,46.9 v36.7,46.9 36.08,47.52 36.08,47.74 35.95,47.88 33.89,47.88 32.59,49.19 | 32.48,49.29 32.59,49.19 | v28.3,50.9 28.8,50.41 30.73,50.41 31.84,49.29 32.48,49.29 | 32.48,49.29 32.59,49.19
  Bottom 0.152: 36.8,46.9 v36.7,46.9 37.01,46.9 38.06,47.95 38.06,48.16 38.82,48.92 39.03,48.92 J1.5 | v28.3,50.9 26.1,48.7 S1.P$4
  other vias: 26.1,46.35
N$5
  Top 0.152: D2.2 R3.2
N$6
  Top 0.152: D1.2 R2.2
N$7
  Top 0.152: U1.58 35.25,46.3 Y1.1
N$8
  Top 0.152: U1.59 34.75,45.5 34.63,45.62 34.3,45.62 34.17,45.76 34.17,46.08 Y1.3
N$10
  Top 0.152: U1.56 36.25,45.5 37.33,46.58 37.33,47.12 36.47,47.88 34.92,49.43 J1.1
N$11
  Top 0.152: R7.1 54.77,38.67 U5.1 52.51,37.93 52.51,36.93 55.6,33.84 55.6,28.8 48.76,21.96 J2.P$7
N$12  (via drill 0.3)
  Top 0.152: U5.14 48.38,39.98 48.72,40.32 48.9,40.32 49.18,40.32 49.46,40.04 49.46,39.77 49.66,39.56 49.66,38.56 v49.92,38.31
  Bottom 0.152: v49.92,38.31 50.24,37.98 50.24,37.3 | 50.24,37.3 50.24,37.24 | 50.24,37.3 50.24,34.12 52.49,31.87 52.49,28.92 48.4,24.82 47.66,24.82 47.17,24.34 47.17,23.59 46.55,22.98 J2.P$6
N$13  (via drill 0.3)
  Top 0.152: U5.13 49.35,40.62 v49.99,39.99
  Bottom 0.152: v49.99,39.99 50,39.98 50,38.98 50.31,38.67 50.55,38.67 50.55,34.25 52.8,32 52.8,28.79 J2.P$5
N$14
  Top 0.152: R8.2 54.52,42.58 U5.7 53.08,42.4 51.91,42.4 51.75,42.57 51.05,42.57 50.56,42.08 50.56,41.02 51.59,40 51.59,34.31 54.1,31.8 54.1,30.44 54.17,30.38 54.17,29.27 51.8,26.9 47.5,26.9 46.22,25.62 J2.P$4
N$15
  Top 0.152: R8.1 54.83,41.92 U5.6 51.96,41.92 51.62,42.26 51.18,42.26 50.87,41.95 50.87,41.15 51.9,40.12 51.9,37.2 | 51.9,37.2 51.9,37.18 | J2.P$3 48.57,26.59 51.93,26.59 54.47,29.14 54.47,30.5 54.41,30.57 54.41,31.93 51.9,34.44 51.9,37.2
N$16  (via drill 0.3)
  Top 0.152: U5.11 48.23,41.92 48.67,42.37 49.5,42.37 49.95,41.91 49.95,40.77 50.53,40.2 v50.53,39.2 | J2.P$2 47.21,27.04 47.37,27.2 48.41,27.2 48.95,27.75 51.36,27.75 53.01,29.4 v53.33,29.4
  Bottom 0.152: v50.53,39.2 50.85,38.87 50.85,34.38 53.1,32.13 53.1,29.63 v53.33,29.4
N$17  (via drill 0.3)
  Top 0.152: v51.06,39.78 51.06,40.1 50.26,40.9 50.26,42.04 49.62,42.67 47.45,42.67 U5.10 | v53.64,30.16 53.41,29.93 53.11,29.93 51.24,28.06 J2.P$1
  Bottom 0.152: v51.06,39.78 51.16,39.68 51.16,34.5 53.41,32.25 53.41,30.4 53.64,30.17 v53.64,30.16
N$18
  Top 0.203: U2.9 27.88,25 C9.1
N$19
  Top 0.152: R1.2 46.02,41.23 46.09,41.23 46.32,41 46.32,34.52 43.16,31.36 J2.GRNN
N$20  (via drill 0.3)
  Top 0.152: R5.2 45.4,38.2 44.89,37.7 v44.89,33.91 v44.9,33.9 | J2.YLWN 42.16,20.7 42.16,20.85 42.65,21.34 44.34,21.34 v44.4,21.4
  Bottom 0.152: v44.9,33.9 44.9,32.9 44.3,32.3 44.3,29.25 44.33,29.22 44.33,28.78 44.3,28.75 44.3,21.5 v44.4,21.4
N$23
  Top 0.203: U6.10 29.57,13.65 29.94,13.65 30.2,13.39 C14.1
OA1  (via drill 0.3)
  Top 0.152: U2.5 25.15,24.31 24.99,24.15 24.99,24.04 24.72,24.04 24.23,23.55 24.23,23.23 23.31,22.3 20.2,22.3 19.34,23.17 15.64,23.17 15.31,23.5 v13.1,23.5
  other vias: 8.6,21.3 8.6,22.6 8.6,23.5 8.6,24.4 8.6,25.8 13.1,21.8 13.2,20.7 13.1,26.4 13.1,25.3 12.2,21.8 12.2,22.6 12.2,23.5 12.2,24.4 12.2,25.3 11.3,21.8 11.3,20.7 11.3,23.5 11.3,26.4 11.3,25.3 10.4,21.8 10.4,22.6 10.4,23.5 10.4,24.4 10.4,25.3 9.5,21.8 9.5,20.7 9.5,23.5 9.5,26.4 9.5,25.3 12.8,28.2 5.4,28.2 0.8,28.1 0.8,26.9 5.7,18.3 12.8,18.3 9.5,22.6 11.3,22.6 13.1,22.6 12.2,20.7 10.4,20.7 11.3,24.4 13.1,24.4 9.5,24.4 10.4,26.4 12.2,26.4
  pour Top (rank 2, no thermals): -0.3,28.6 20,28.6 20,17.8 5.2,17.8 5.2,26.4 -0.3,26.4
  pour Bottom (rank 2, no thermals): -0.3,28.6 20,28.6 20,17.8 5.2,17.8 5.2,26.4 -0.3,26.4
OA2  (via drill 0.3)
  Top 0.152: v22.57,15.12 22.89,15.12 25.3,17.53 25.3,21.84 v25.06,22.07 | U2.4 24.65,24.39 24.6,24.34 | 24.6,24.34 | 23.93,23.67 | 23.93,23.67 v23.7,23.45 | 24.6,24.34 23.93,23.67 | v19.3,15.06 19.04,15.06 18.59,15.51 15.55,15.51 15.39,15.35 13.65,15.35 v13.2,15.8
  Bottom 0.152: v19.3,15.06 19.54,15.06 20,14.61 22,14.61 22.52,15.12 v22.57,15.12 | v23.7,23.45 23.7,23.43 23.91,23.22 23.93,23.22 24.54,22.61 24.54,22.59 v25.06,22.07
  other vias: 8.7,11.7 8.7,13.1 8.7,14 8.7,14.9 8.7,16.3 13.2,12.3 13.2,11.2 13.2,14 5.7,17.1 12.3,12.3 12.3,13.1 12.3,14 12.3,14.9 12.3,15.8 11.4,12.3 11.4,11.2 11.4,14 11.4,16.8 11.4,15.8 10.5,12.3 10.5,13.1 10.5,14 10.5,14.9 10.5,15.8 9.6,12.3 9.6,11.2 9.6,14 9.6,16.8 9.6,15.8 0.8,25.6 4.5,23.5 1,15.7 0.8,8.3 13.2,16.8 13.7,8.9 10.4,5.8 9.6,13.1 11.4,13.1 13.2,13.1 13.2,14.9 11.4,14.9 9.6,14.9 10.5,16.8 12.3,16.8 12.3,11.2 10.5,11.2
  pour Top (rank 4, no thermals): -0.3,26.1 4.9,26.1 4.9,17.5 20,17.5 20,-1.5 -0.3,-1.5
  pour Bottom (rank 4, no thermals): -0.3,26.1 4.9,26.1 4.9,17.5 20,17.5 20,-1.1 -0.3,-1.1
OB1  (via drill 0.3)
  Top 0.152: v25.4,33.2 24.8,33.2 24.38,33.62 24.38,33.94 24.06,34.25 24.06,34.95 24.3,35.18 24.3,37.61 23.2,38.71 21.05,40.85 20.41,41.52 20.41,41.53 20.32,41.61 20.23,41.7 19.44,42.49 15.91,42.49 15.4,43 13.2,43 v13.1,42.9 | U2.20 25.15,30.05 24.95,30.25 24.95,30.94 v25.18,31.17
  Bottom 0.152: v25.4,33.2 25.4,31.39 v25.18,31.17
  other vias: 8.6,40.7 8.6,42 8.6,42.9 8.6,43.8 8.6,45.2 13.1,41.2 13.1,45.8 13.1,44.7 12.2,41.2 12.2,42 12.2,42.9 12.2,43.8 12.2,44.7 11.3,41.2 11.3,40.2 11.3,42.9 11.3,45.8 11.3,44.7 10.4,41.2 10.4,42 10.4,42.9 10.4,43.8 10.4,44.7 9.5,41.2 9.5,40.2 9.5,42.9 9.5,45.8 9.5,44.7 0.8,31.9 4.5,34.1 5.7,39.9 1.3,40.8 2.5,48.2 13.1,40.2 12.7,50.3 11.2,48.9 9.5,43.8 11.3,43.8 13.1,43.8 12.2,45.8 10.4,45.8 10.4,40.2 12.2,40.2 9.5,42 11.3,42 13.1,42
  pour Top (rank 3, no thermals): -0.3,31.5 5,31.5 5,39.5 19.7,39.5 19.5,58.3 -0.5,58.3
  pour Bottom (rank 3, no thermals): -0.3,31.5 5,31.5 5,39.5 20,39.5 20,57.7 -0.3,57.7
OB2  (via drill 0.3)
  Top 0.152: v17.3,33.7 v17.31,33.71 16.77,33.17 15.64,33.17 15.39,33.42 13.18,33.42 v13.1,33.5 | v22.7,33.3 22.93,33.07 22.93,32.67 23.54,32.06 24.34,32.06 24.65,31.75 U2.21
  Bottom 0.152: v17.31,33.71 17.81,33.71 20,35.9 20.47,35.9 22.17,34.2 22.17,33.88 22.7,33.35 v22.7,33.3
  other vias: 8.6,31.2 8.6,32.6 8.6,33.5 8.6,34.4 8.6,35.8 13.1,31.8 13.1,30.7 13,36.3 13.1,35.3 12.2,31.8 12.2,32.6 12.2,33.5 12.2,34.4 12.2,35.3 11.3,31.8 11.3,30.7 11.3,33.5 11.3,36.3 11.3,35.3 10.4,31.8 10.4,32.6 10.4,33.5 10.4,34.4 10.4,35.3 9.5,31.8 9.5,30.7 9.5,33.5 9.5,36.3 9.5,35.3 5.7,38.7 0.8,29.4 0.8,30.8 5.4,29.3 12.8,29.4 12.8,38.7 9.5,34.4 11.3,34.4 13.1,34.4 9.5,32.6 11.3,32.6 13.1,32.6 10.4,30.7 12.2,30.7 10.4,36.3 12.2,36.3
  pour Top (rank 2, no thermals): -0.3,29 20,29 20,39.2 5.2,39.2 5.2,31.2 -0.3,31.2
  pour Bottom (rank 2, no thermals): -0.3,29 20,29 20,39.2 5.2,39.2 5.2,31.2 -0.3,31.2
RTD
  Top 0.152: U4.2 13.04,49.1 13.77,48.36 17.34,48.36 19.63,46.07 20.12,46.07 22.22,48.17 29.8,48.17 30.48,47.49 30.48,46.98 29,45.5 R6.2 30.45,44.25 30.95,43.75 U1.2
SRA  (via drill 0.3)
  Top 0.152: R13.2 21.3,19.1 22.5,19.1 22.9,19.5 22.9,21.4 23.2,21.7 23.56,21.7 24.75,22.88 v25.07,22.88 | v26.13,23.2 26.13,24 26.65,24.52 U2.8
  Bottom 0.152: v25.07,22.88 25.39,23.2 v26.13,23.2
  pour Top (no thermals): 14,13.2 18.5,13.2 19.9,14.6 19.9,18.2 17.4,20.8 14,20.8 14,22.7 22.1,22.7 22.1,13.5 19.8,11.4 14,11.4
SRB  (via drill 0.3)
  Top 0.152: R12.2 22.5,37 v23.4,36.1 | v24.9,34.6 26.65,32.85 U2.17
  Bottom 0.152: v23.4,36.1 v24.9,34.6
  pour Top (no thermals): 13.9,32.6 18.4,32.6 20.2,34.5 20.2,38.3 18.3,40.2 13.9,40.2 13.9,41.9 19.1,41.9 22.2,38.8 22.1,30.8 13.9,30.8
STLCLK  (via drill 0.3)
  Top 0.152: R3.1 19.98,51.04 19.98,50.55 20.73,49.8 30.47,49.8 32.33,47.94 v32.33,47.7 | v37.9,47 37.64,46.74 37.64,46.45 36.75,45.56 U1.55
  Bottom 0.152: v32.33,47.7 32.53,47.5 34.9,47.5 35.4,47 35.4,45.8 36.7,45.8 v37.9,47
STLERR  (via drill 0.3)  (1 unrouted)
  Top 0.152: v32.26,48.76 32.1,48.6 30.6,50.1 23.45,50.1 R2.1 | v38.44,47.53 38.44,46.78 38.12,46.47 38.09,46.47 37.25,45.63 U1.54
  Bottom 0.152: v32.26,48.76 33.22,47.8 35.03,47.8 35.32,47.52 36.98,47.52 38.51,49.04 38.52,49.05 38.52,49.67 39.17,50.32 39.91,50.32 40.43,49.8 40.43,49.06 39.91,48.54 39.17,48.54 39.09,48.62 38.95,48.62 38.37,48.03 38.37,47.6 v38.44,47.53
TMC_CSN
  Top 0.152: U2.14 27.45,28.15 28.45,27.14 31.61,27.14 32.38,27.91 32.38,31.05 33.85,32.52 J8.5 33.75,33.51 U1.20
TMC_DIR  (via drill 0.3)
  Top 0.152: U2.30 21.86,26.65 v21.84,26.62 | v18.68,33.58 18.68,33.9 18.63,33.95 18.63,34.43 18.81,34.61 18.81,35.07 19.04,35.29 19.04,37.51 18.81,37.73 18.81,38.24 18.63,38.41 v18.63,39.17 | v19.8,48.11 20.33,48.65 20.33,48.83 20.69,49.19 30.22,49.19 31.5,47.91 31.5,46.67 32.25,45.92 U1.64
  Bottom 0.152: v21.84,26.62 21.84,26.66 21.31,27.18 21.31,27.53 21.01,27.83 21.01,28.15 19.04,30.13 19.04,33.22 v18.68,33.58 | v18.63,39.17 19.04,39.58 19.04,46.21 19.01,46.23 19.01,47.22 19.8,48.01 v19.8,48.11
TMC_EN
  Top 0.152: U2.15 27.45,28.65 27.73,28.37 27.73,28.3 28.58,27.45 31.49,27.45 32.07,28.03 32.07,31.18 32.6,31.7 32.6,33.9 33.25,34.55 33.25,34.8 | 33.25,34.8 U1.19 | R9.1 31.35,34.8 33.25,34.8
TMC_MISO
  Top 0.152: U2.10 27.77,26.15 27.77,26.23 33.41,26.23 33.82,25.82 | 33.82,25.82 J8.2 | U1.22 34.75,34.59 35.32,34.02 35.32,27.32 33.82,25.82
TMC_MOSI  (via drill 0.3)
  Top 0.152: U2.11 28.05,26.65 28.17,26.53 32.53,26.53 33.85,27.85 J8.3 | U1.23 35.25,34.85 v35.3,34.8
  Bottom 0.152: v35.3,34.8 35.3,29.78 J8.3
TMC_SCK
  Top 0.152: U2.12 27.35,27 28.13,27 28.29,26.84 31.74,26.84 32.68,27.78 32.68,29.7 J8.4 35.02,32.04 35.02,33.89 34.25,34.66 U1.21
TMC_SG  (via drill 0.3)
  Top 0.152: U2.27 21.95,28.15 v21.9,28.2 | v19.7,34.7 v19.7,38.1 | v19.9,46.6 20.33,47.03 20.33,48.21 20.64,48.52 20.64,48.7 20.81,48.88 30.09,48.88 31.19,47.78 31.19,46.55 31.5,46.24 U1.1
  Bottom 0.152: v21.9,28.2 19.7,30.4 v19.7,34.7 | v19.7,38.1 19.7,46.4 v19.9,46.6
TMC_STEP  (via drill 0.3)
  Top 0.152: v18.14,33.04 18.14,33.84 18.33,34.03 18.33,34.56 18.51,34.74 18.51,35.19 18.73,35.42 18.73,37.38 18.51,37.61 18.51,38.11 18.33,38.29 18.33,38.72 18.1,38.95 18.1,39.6 v18.04,39.66 | v19.8,48.87 20.42,49.49 30.35,49.49 31.8,48.04 31.8,46.8 32.75,45.85 U1.63 | U2.31 22.13,26.15 v21.84,25.87
  Bottom 0.152: v21.84,25.87 21.62,26.09 21.61,26.09 21.41,26.3 21.4,26.3 21.3,26.4 21.3,26.76 21.01,27.05 21.01,27.41 20.71,27.71 20.71,28.03 18.73,30 18.73,32.8 18.49,33.04 v18.14,33.04 | v18.04,39.66 18.29,39.66 18.73,40.1 18.73,46.08 18.71,46.11 18.71,47.35 19.27,47.91 19.27,48.33 v19.8,48.87
V+  (via drill 0.3)
  Top 0.203: U6.11 29.49,14.23 v30.14,14.23
  Top 0.254: v35.3,7.9 35.7,8.3 41.76,8.3 43.36,6.7 46.4,6.7 49.22,9.52 49.52,9.52 51.76,11.77 J3.2
  Top 0.305: U2.25 21.75,29.15 21.61,29 21.61,28.97 21.43,28.8 21.39,28.8 C12.1 19.3,29.7 C8.2 18.55,29.2 v18.2,29.2 v17.4,29.2
  Bottom 0.203: v30.14,14.23 30.14,11.64 v28.5,10
  Bottom 0.254: v35.3,7.9 28.6,7.9 v28.5,8
  other vias: 15.8,35.3 15.8,44.3 16,14.9 16,23.9 16.6,34.6 15.8,34.6 15.9,43.4 16,14.1 16.8,14.9 16.8,14.1 18.2,14.9 18.2,14.1 16,24.7 16.8,24.7 16.8,23.9 19,23.9 19,24.7 17.6,35.3 16.8,43.1 17.2,44.3 18,43.1 16,33.8 16.5,43.8 17.4,34.6 28.5,9 28.5,7 28.5,6 28.5,5 28.5,4 28.5,3 28.5,2 28.5,1
  pour Bottom: 14.5,-0.5 29.2,-0.5 29.2,10.8 19.6,10.8 19.5,57.5 14.5,57.5
  pour Top (rank 2, no thermals): 19.1,15.4 14,15.4 14,13.5 18.4,13.5 19.1,14.2
  pour Top (no thermals): 19.7,25.2 14,25.2 14,23.3 19.7,23.3
  pour Top (no thermals): 18.3,35.6 13.9,35.6 13.9,33 18.3,33
  pour Top (no thermals): 17.4,44.7 13.9,44.7 13.9,42.7 19.4,42.7
  pour Top (no thermals): 26.4,10.6 30.4,10.6 30.4,-0.3 26.4,-0.3
  pour Top (no thermals): 26.9,14.4 25.7,14.4 25.3,14.4 24.9,14 24.9,12 26.4,10.5 27.3,10.5 25.5,12.3 25.5,13.5 25.6,13.6 25.8,13.6 26.9,13.6
VSW
  pour Top (no thermals): 26.1,14.7 26.1,15.8 26.9,16.6 29.4,16.6 30.3,17.5 32.2,17.5 32.2,11 30.5,11 30.5,14.2 30.1,14.6 29.1,14.6 29.1,15.1 28.6,15.1 28.6,16 27.4,16 27.4,15.1 27,15.1 26.9,15.1 26.9,14.7

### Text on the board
tPlace: PDI | pwr | clk | err | atkstepper23 v0.32 | rst | B1 | B2 | A1 | spi | A2 | ATXP0 | 24v - GND | V+ | GND
bPlace: His speech was full of mutterings, warnings. / The artist's life is strewn with traps. / Beware "the machinations of the enemy." / "Mr. Lytle", I whispered, "who is the enemy?" / He sat up. His unfocused eyes were an icy blue. / "Why, boy," he said, "the bourgeoisie!" / Then he peered at me for a second as if he'd forgotten who I was. / "Of course," he said. / "You're only a baby."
